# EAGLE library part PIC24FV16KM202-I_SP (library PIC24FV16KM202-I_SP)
MICROCHIP - PIC24FV16KM202-I/SP - MCU, 16BIT, PIC24, 32MHZ, SPDIP-28 Source: Datasheet
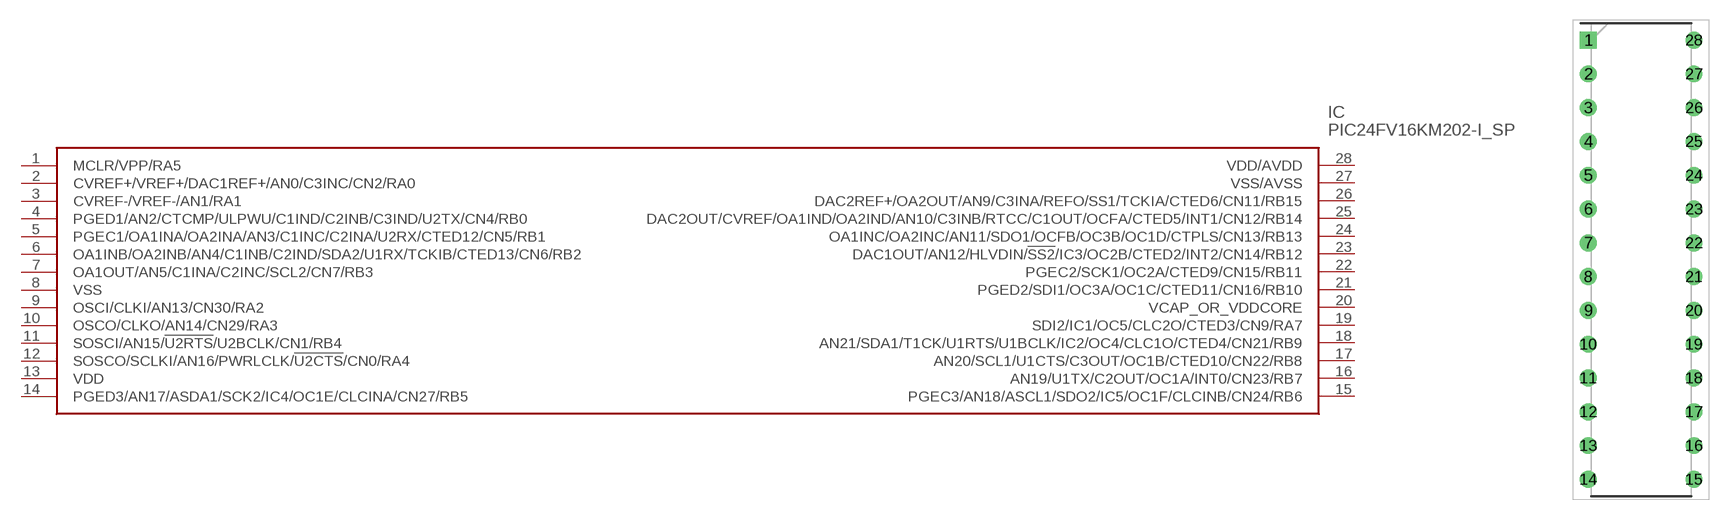
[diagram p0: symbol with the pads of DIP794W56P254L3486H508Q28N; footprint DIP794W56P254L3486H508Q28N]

Designator prefix IC

## PIC24FV16KM202-I_SP (Allied_Number: 70451531; Allied_Price-Stock: https://www.alliedelec.com/microchip-technology-inc-pic24fv16km202-i-sp/70451531/; Description: MICROCHIP - PIC24FV16KM202-I/SP - MCU, 16BIT, PIC24, 32MHZ, SPDIP-28; Height: 5.08mm; Manufacturer_Name: Microchip; Manufacturer_Part_Number: PIC24FV16KM202-I/SP; Mouser_Part_Number: 579-24FV16KM202I/SP; Mouser_Price-Stock: https://www.mouser.com/Search/Refine.aspx?Keyword=579-24FV16KM202I%2FSP; RS_Part_Number: 1772530; RS_Price-Stock: http://uk.rs-online.com/web/p/products/1772530)  [DIP794W56P254L3486H508Q28N]
1  MCLR/VPP/RA5
2  CVREF+/VREF+/DAC1REF+/AN0/C3INC/CN2/RA0
3  CVREF-/VREF-/AN1/RA1
4  PGED1/AN2/CTCMP/ULPWU/C1IND/C2INB/C3IND/U2TX/CN4/RB0
5  PGEC1/OA1INA/OA2INA/AN3/C1INC/C2INA/U2RX/CTED12/CN5/RB1
6  OA1INB/OA2INB/AN4/C1INB/C2IND/SDA2/U1RX/TCKIB/CTED13/CN6/RB2
7  OA1OUT/AN5/C1INA/C2INC/SCL2/CN7/RB3
8  VSS  pwr
9  OSCI/CLKI/AN13/CN30/RA2
10  OSCO/CLKO/AN14/CN29/RA3
11  SOSCI/AN15/!U2RTS!/U2BCLK/CN1/RB4
12  SOSCO/SCLKI/AN16/PWRLCLK/!U2CTS!/CN0/RA4
13  VDD  pwr
14  PGED3/AN17/ASDA1/SCK2/IC4/OC1E/CLCINA/CN27/RB5
15  PGEC3/AN18/ASCL1/SDO2/IC5/OC1F/CLCINB/CN24/RB6
16  AN19/U1TX/C2OUT/OC1A/INT0/CN23/RB7
17  AN20/SCL1/U1CTS/C3OUT/OC1B/CTED10/CN22/RB8
18  AN21/SDA1/T1CK/U1RTS/U1BCLK/IC2/OC4/CLC1O/CTED4/CN21/RB9
19  SDI2/IC1/OC5/CLC2O/CTED3/CN9/RA7
20  VCAP_OR_VDDCORE
21  PGED2/SDI1/OC3A/OC1C/CTED11/CN16/RB10
22  PGEC2/SCK1/OC2A/CTED9/CN15/RB11
23  DAC1OUT/AN12/HLVDIN/!SS2!/IC3/OC2B/CTED2/INT2/CN14/RB12
24  OA1INC/OA2INC/AN11/SDO1/OCFB/OC3B/OC1D/CTPLS/CN13/RB13
25  DAC2OUT/CVREF/OA1IND/OA2IND/AN10/C3INB/RTCC/C1OUT/OCFA/CTED5/INT1/CN12/RB14
26  DAC2REF+/OA2OUT/AN9/C3INA/REFO/SS1/TCKIA/CTED6/CN11/RB15
27  VSS/AVSS  pwr
28  VDD/AVDD  pwr

## Footprint DIP794W56P254L3486H508Q28N (pad centres in mm)
28-Lead Skinny Plastic Dual In-Line (SP) - 300mil Body [SPDIP]
drill 0.759 pad 1.159 square: 1 -3.969,16.51
drill 0.759 pad 1.159: 2 -3.969,13.97; 3 -3.969,11.43; 4 -3.969,8.89; 5 -3.969,6.35; 6 -3.969,3.81; 7 -3.969,1.27; 8 -3.969,-1.27; 9 -3.969,-3.81; 10 -3.969,-6.35; 11 -3.969,-8.89; 12 -3.969,-11.43; 13 -3.969,-13.97; 14 -3.969,-16.51; 15 3.969,-16.51; 16 3.969,-13.97; 17 3.969,-11.43; 18 3.969,-8.89; 19 3.969,-6.35; 20 3.969,-3.81; 21 3.969,-1.27; 22 3.969,1.27; 23 3.969,3.81; 24 3.969,6.35; 25 3.969,8.89; 26 3.969,11.43; 27 3.969,13.97; 28 3.969,16.51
